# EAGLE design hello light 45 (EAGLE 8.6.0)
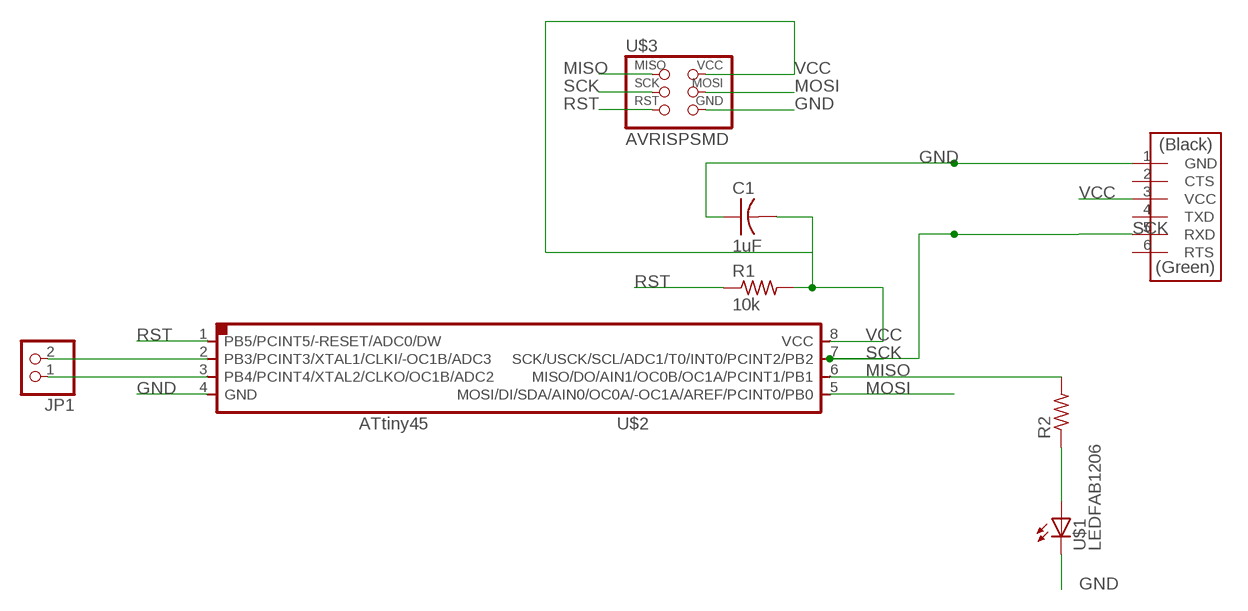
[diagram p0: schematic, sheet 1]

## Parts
C1  1uF  CAP-US1206FAB  [C1206FAB]
JP1  PINHD-1X2  [1X02]
R1  10k  RES-US1206FAB  [R1206FAB]
R2  RES-US1206FAB  [R1206FAB]
U$1  LEDFAB1206  [LED1206FAB]
U$2  ATTINY45SI  [SOIC8]
U$3  AVRISPSMD  [2X03SMD]
U$4  FTDI-SMD-HEADER  [1X06SMD]

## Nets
GND: C1.1 U$1.2(C) U$2.4(GND) U$3.6(GND) U$4.1(GND)
MISO: R2.2 U$2.6(MISO/DO/AIN1/OC0B/OC1A/PCINT1/PB1) U$3.1(MISO)
MOSI: U$2.5(MOSI/DI/SDA/AIN0/OC0A/-OC1A/AREF/PCINT0/PB0) U$3.4(MOSI)
N$1: R2.1 U$1.1(A)
N$2: JP1.2 U$2.2(PB3/PCINT3/XTAL1/CLKI/-OC1B/ADC3)
N$3: JP1.1 U$2.3(PB4/PCINT4/XTAL2/CLKO/OC1B/ADC2)
RST: R1.1 U$2.1(PB5/PCINT5/-RESET/ADC0/DW) U$3.5(RST)
SCK: U$2.7(SCK/USCK/SCL/ADC1/T0/INT0/PCINT2/PB2) U$3.3(SCK) U$4.5(RXD)
VCC: C1.2 R1.2 U$2.8(VCC) U$3.2(VCC) U$4.3(VCC)
Unconnected: U$4.2(CTS) U$4.4(TXD) U$4.6(RTS)

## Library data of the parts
C1 = fab:CAP-US
JP1 = pinhead:PINHD-1X2: PIN HEADER
R1 R2 = fab:RES-US: Resistor (US Symbol)
U$1 = fab:LED: LED
U$2 = fab:ATTINY45
U$3 = fab:AVRISP
U$4 = fab:FTDI-SMD-HEADER

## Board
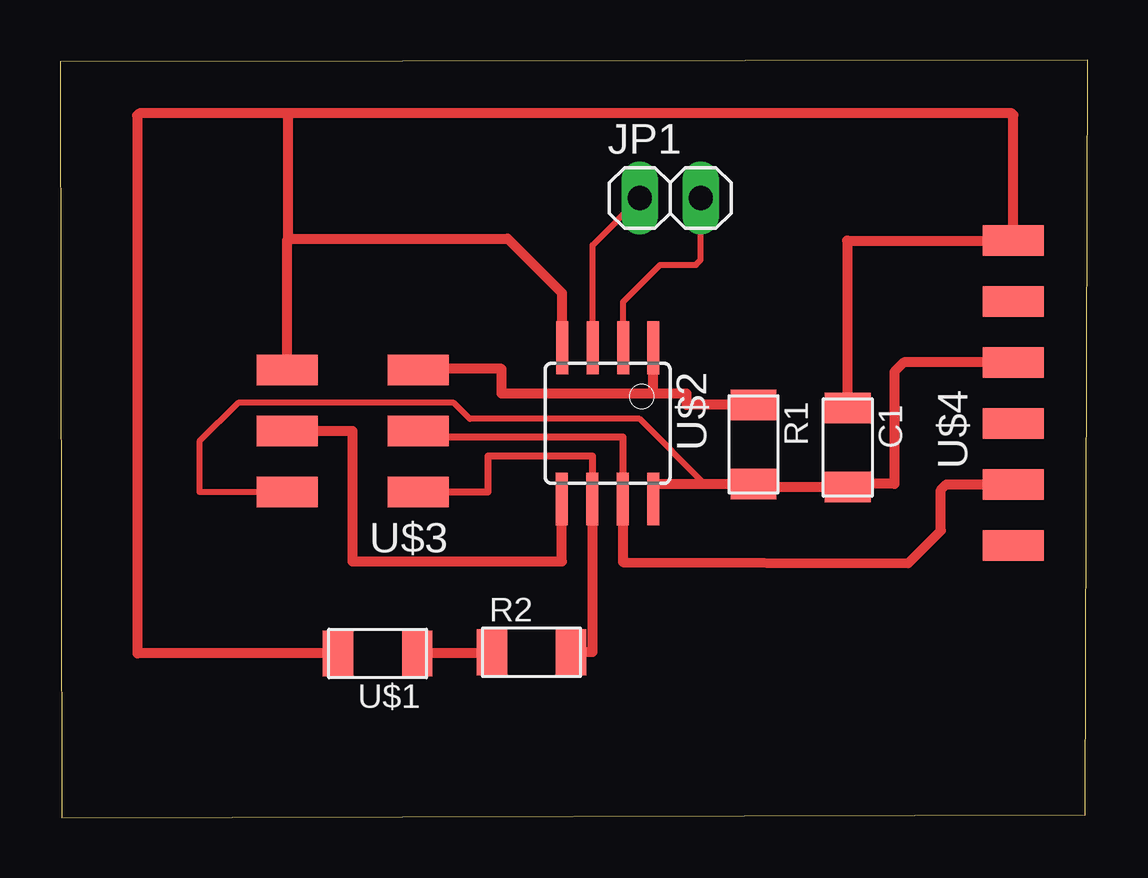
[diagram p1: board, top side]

Size 42.81 x 31.58 mm. Coordinates in mm from the lower left corner, seen from the top.
Outline: 0.07,0 42.72,0.13 42.81,31.58 0,31.51 0.07,0
Copper layers (1*16): Top 0.035mm / dielectric 1.5mm / Bottom 0.035mm
Design rules "default *": minimum track width 10mil, minimum drill 24mil, track to track 16mil, track to pad 16mil, pad to pad 16mil, via to via 16mil, smd to smd 16mil, copper to edge 40mil, drill to drill 8mil, minimum pad ring 10mil, minimum via ring 8mil, stop-mask expansion 4mil, vias tented up to drill 0mil, thermal gap 10mil

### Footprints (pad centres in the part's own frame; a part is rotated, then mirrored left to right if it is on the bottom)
C1206FAB = smd 1.27 x 1.905: 1 -1.651,0; 2 1.651,0
1X02 = drill 1.016 long: 1 -1.27,0; 2 1.27,0
R1206FAB = smd 1.27 x 1.905: 1 -1.651,0; 2 1.651,0
LED1206FAB = smd 1.27 x 1.905: 1 -1.651,0; 2 1.651,0
SOIC8 = smd 0.5 x 2.2: 1 -1.905,-3.154; 2 -0.645,-3.154; 3 0.625,-3.154; 4 1.895,-3.154; 5 1.905,3.154; 6 0.635,3.154; 7 -0.635,3.154; 8 -1.905,3.154
2X03SMD = smd 2.54 x 1.27: 1 -2.54,2.54; 2 2.92,2.54; 3 -2.54,0; 4 2.92,0; 5 -2.54,-2.54; 6 2.92,-2.54
1X06SMD = smd 2.54 x 1.27: 1 0,6.35; 2 0,3.81; 3 0,1.27; 4 0,-1.27; 5 0,-3.81; 6 0,-6.35

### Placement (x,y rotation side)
C1  32.82,15.43 270 top
JP1  25.43,25.83 0 top
R1  28.89,15.56 270 top
R2  19.65,6.9 0 top
U$1  13.23,6.85 180 top
U$2  22.82,16.44 180 top
U$3  12.38,16.13 180 top
U$4  39.72,17.71 0 top

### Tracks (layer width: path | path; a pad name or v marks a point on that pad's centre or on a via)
GND
  Top 0.406: 39.38,24.4 U$4.1 | 32.8,24.06 32.8,24.05 | 32.8,24.05 32.8,17.11 C1.1 | U$3.6 9.46,24.06 9.51,24.11 | U$1.2 3.23,6.85 3.23,29.24 3.21,29.26 3.31,29.36 9.51,29.36 | U$4.1 39.72,29.29 39.66,29.36 9.51,29.36 | 9.51,24.11 9.51,29.36 | 32.8,24.05 U$4.1 | U$2.4 20.92,21.87 18.65,24.14 18.62,24.11 9.51,24.11
MISO
  Top 0.3: U$3.1 17.84,13.59 17.84,15.08 22.18,15.08 U$2.6
  Top 0.406: 22.18,13.22 U$2.6 22.18,6.9 R2.2 | 14.92,13.56 U$3.1
MOSI
  Top 0.406: U$3.4 12.18,16.13 12.18,10.69 20.91,10.69 U$2.5
N$1
  Top 0.406: R2.1 18,6.85 U$1.1
N$2
  Top 0.254: U$2.2 23.46,21.5 25.01,23.05 26.5,23.05 26.7,23.25 JP1.2
N$3
  Top 0.254: U$2.3 22.19,23.87 JP1.1
RST
  Top 0.406: R1.1 26.1,17.21 26.1,17.68 24.74,17.68 | 24.74,17.68 18.4,17.68 18.4,18.7 14.92,18.7 U$3.5 | 24.74,17.68 24.72,17.68 U$2.1
SCK
  Top 0.3: U$3.3 15.94,16.13 15.94,15.88 23.45,15.88 U$2.7
  Top 0.406: U$2.7 23.45,10.65 35.35,10.62 36.71,11.97 36.71,13.67 36.93,13.9 U$4.5 | 14.92,15.88 U$3.3
VCC
  Top 0.254: R1.2 26.87,13.91 24.15,16.63 17.08,16.63 16.41,17.3 7.42,17.3 5.8,15.68 5.8,13.59 U$3.2
  Top 0.406: U$4.3 35.16,18.98 34.77,18.58 34.77,13.91 32.95,13.91 C1.2 28.89,13.78 R1.2 24.72,13.91 U$2.8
